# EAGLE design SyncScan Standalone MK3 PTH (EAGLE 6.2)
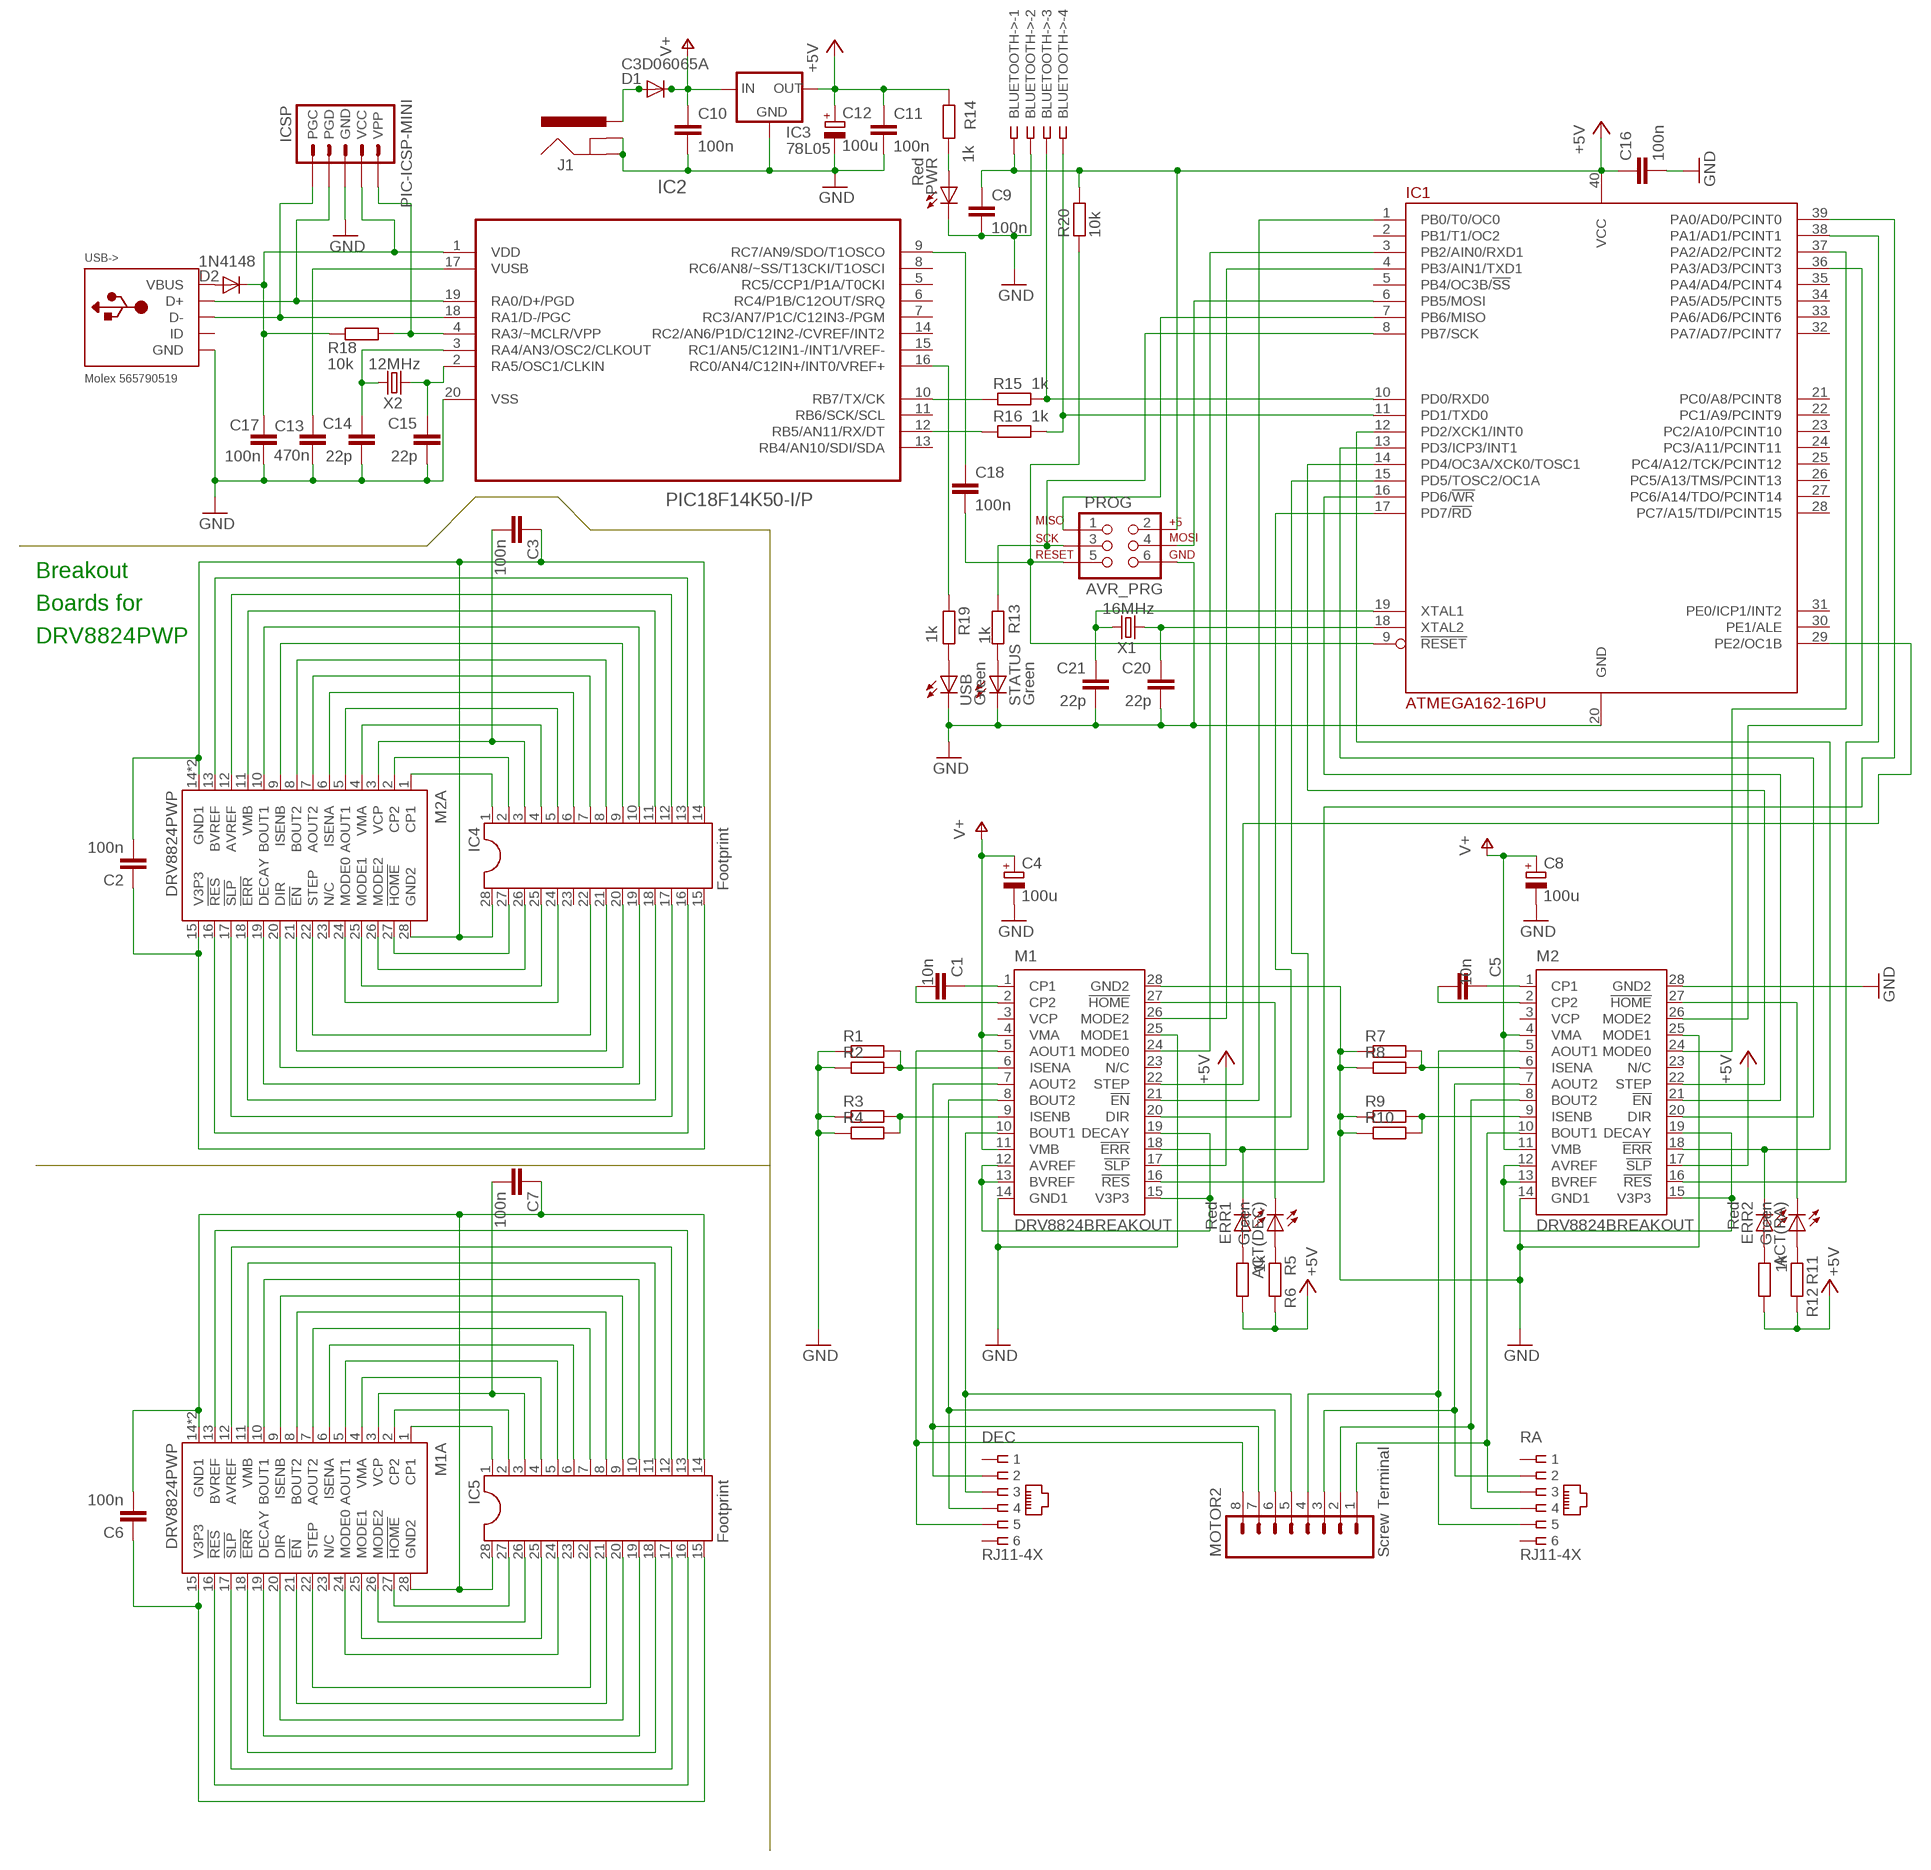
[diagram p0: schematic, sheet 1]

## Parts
ACT(DEC)  Green  LED3MM  [LED3MM]
ACT(RA)  Green  LED3MM  [LED3MM]
BLUETOOTH->  http://www.ebay.co.uk/itm/250991624201  SSW-104-02-S-S-RA  [SSW-104-02-S-S-RA]
C1  10n  C-EU025-024X044  [C025-024X044]
C2  100n  C-EUC0603K  [C0603K]
C3  100n  C-EUC0603K  [C0603K]
C4  100u  CPOL-EUE2.5-6  [E2,5-6]
C5  10n  C-EU025-024X044  [C025-024X044]
C6  100n  C-EUC0603K  [C0603K]
C7  100n  C-EUC0603K  [C0603K]
C8  100u  CPOL-EUE2.5-6  [E2,5-6]
C9  100n  C-EU025-024X044  [C025-024X044]
C10  100n  C-EU025-024X044  [C025-024X044]
C11  100n  C-EU025-024X044  [C025-024X044]
C12  100u  CPOL-EUE2.5-6  [E2,5-6]
C13  470n  C-EU025-024X044  [C025-024X044]
C14  22p  C-EU025-024X044  [C025-024X044]
C15  22p  C-EU025-024X044  [C025-024X044]
C16  100n  C-EU025-024X044  [C025-024X044]
C17  100n  C-EU025-024X044  [C025-024X044]
C18  100n  C-EU025-024X044  [C025-024X044]
C20  22p  C-EU025-024X044  [C025-024X044]
C21  22p  C-EU025-024X044  [C025-024X044]
D1  C3D06065A  BYW80  [TO220ACS]
D2  1N4148  DIODE1N4148  [DIODE-1N4148]
DEC  RJ11-4X  [RJ11-NO_SHIELD]
ERR1  Red  LED3MM  [LED3MM]
ERR2  Red  LED3MM  [LED3MM]
IC1  ATMEGA162-16PU  [DIL40]
IC2  PIC18F14K50-I/P  [DIL20]
IC3  78L05  V_REG_78XXTO-92  [TO-92]
IC4  Footprint  DIL28  [DIL28-6]
IC5  Footprint  DIL28  [DIL28-6]
ICSP  PIC-ICSP-MINI  [PIC-ICSP-MINI]
J1  POWER_JACKPTH  [POWER_JACK_PTH]
M1  DRV8824BREAKOUT  [DIL28-6]
M1A  DRV8824PWP  [HTSSOP28PWP]
M2  DRV8824BREAKOUT  [DIL28-6]
M2A  DRV8824PWP  [HTSSOP28PWP]
MOTOR2  Screw Terminal  M083.5MM-8  [SCREWTERMINAL-3.5MM-8]
PROG  AVR_PRG  AVR_SPI_PRG_6PTH  [2X3]
PWR  Red  LED3MM  [LED3MM]
R1  1.5R  R-EU_0309/12  [0309/12]
R2  1.5R  R-EU_0309/12  [0309/12]
R3  1.5R  R-EU_0309/12  [0309/12]
R4  1.5R  R-EU_0309/12  [0309/12]
R5  1k  R-EU_0204/7  [0204/7]
R6  1k  R-EU_0204/7  [0204/7]
R7  1.5R  R-EU_0309/12  [0309/12]
R8  1.5R  R-EU_0309/12  [0309/12]
R9  1.5R  R-EU_0309/12  [0309/12]
R10  1.5R  R-EU_0309/12  [0309/12]
R11  1k  R-EU_0204/7  [0204/7]
R12  1k  R-EU_0204/7  [0204/7]
R13  1k  R-EU_0204/7  [0204/7]
R14  1k  R-EU_0204/7  [0204/7]
R15  1k  R-EU_0204/7  [0204/7]
R16  1k  R-EU_0204/7  [0204/7]
R18  10k  R-EU_0204/7  [0204/7]
R19  1k  R-EU_0204/7  [0204/7]
R20  10k  R-EU_0204/7  [0204/7]
RA  RJ11-4X  [RJ11-NO_SHIELD]
STATUS  Green  LED3MM  [LED3MM]
USB  Green  LED3MM  [LED3MM]
USB->  Molex 565790519  USBMOLEX  [USB-MINIB-THM-MOLEX]
X1  16MHz  CRYSTALHC49US  [HC49US]
X2  12MHz  CRYSTALHC49US  [HC49US]

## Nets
3.3V-1: M1.12(AVREF) M1.13(BVREF) M1.15(V3P3) M1.19(DECAY)
3.3V-2: M2.12(AVREF) M2.13(BVREF) M2.15(V3P3) M2.19(DECAY)
!EN: IC4.21 M2A.21(!EN)
!EN1: IC5.21 M1A.21(!EN)
!EN-1: IC1.1(PB0/T0/OC0) M1.21(!EN)
!EN-2: IC1.16(PD6/!WR) M2.21(!EN)
!ERR: IC4.18 M2A.18(!ERR)
!ERR1: IC5.18 M1A.18(!ERR)
!ERR-1: ERR1.K(C) IC1.15(PD5/TOSC2/OC1A) M1.18(!ERR)
!ERR-2: ERR2.K(C) IC1.12(PD2/XCK1/INT0) M2.18(!ERR)
!HOME: IC4.27 M2A.27(!HOME)
!HOME1: IC5.27 M1A.27(!HOME)
!HOME-1: ACT(DEC).K(C) M1.27(!HOME)
!HOME-2: ACT(RA).K(C) M2.27(!HOME)
!RES: IC4.16 M2A.16(!RES)
!RES1: IC5.16 M1A.16(!RES)
!RST-1: IC1.39(PA0/AD0/PCINT0) M1.16(!RES)
!RST-2: IC1.38(PA1/AD1/PCINT1) M2.16(!RES)
!SLP: IC4.17 M2A.17(!SLP)
!SLP1: IC5.17 M1A.17(!SLP)
+5V: BLUETOOTH->.1 C9.1 C11.1 C12.+ C16.1 IC1.40(VCC) IC3.1(OUT) M1.17(!SLP) M2.17(!SLP) PROG.2 R5.2 R6.2 R11.2 R12.2 R14.1 R20.2
A1-1: DEC.5 M1.5(AOUT1) MOTOR2.8
A1-2: M2.5(AOUT1) MOTOR2.4 RA.5
A2-1: DEC.2 M1.7(AOUT2) MOTOR2.7
A2-2: M2.7(AOUT2) MOTOR2.3 RA.2
AOUT1: IC4.5 M2A.5(AOUT1)
AOUT2: IC4.7 M2A.7(AOUT2)
AOUT3: IC5.5 M1A.5(AOUT1)
AOUT4: IC5.7 M1A.7(AOUT2)
AVREF: IC4.12 M2A.12(AVREF)
AVREF1: IC5.12 M1A.12(AVREF)
AVROSC1: C21.1 IC1.19(XTAL1) X1.2
AVROSC2: C20.1 IC1.18(XTAL2) X1.1
B1-1: DEC.3 M1.10(BOUT1) MOTOR2.5
B1-2: M2.10(BOUT1) MOTOR2.1 RA.3
B2-1: DEC.4 M1.8(BOUT2) MOTOR2.6
B2-2: M2.8(BOUT2) MOTOR2.2 RA.4
BOUT1: IC4.10 M2A.10(BOUT1)
BOUT2: IC4.8 M2A.8(BOUT2)
BOUT3: IC5.8 M1A.8(BOUT2)
BOUT4: IC5.10 M1A.10(BOUT1)
BVREF: IC4.13 M2A.13(BVREF)
BVREF1: IC5.13 M1A.13(BVREF)
CP1: IC4.1 M2A.1(CP1)
CP1-1: C1.1 M1.1(CP1)
CP1-2: C5.1 M2.1(CP1)
CP2: IC4.2 M2A.2(CP2)
CP2-1: C1.2 M1.2(CP2)
CP2-2: C5.2 M2.2(CP2)
CP3: IC5.1 M1A.1(CP1)
CP4: IC5.2 M1A.2(CP2)
D+: IC2.19(RA0/D+/PGD) ICSP.4(PGD) USB->.D+
D-: IC2.18(RA1/D-/PGC) ICSP.5(PGC) USB->.D-
DECAY: IC4.19 M2A.19(DECAY)
DECAY1: IC5.19 M1A.19(DECAY)
DIR: IC4.20 M2A.20(DIR)
DIR1: IC5.20 M1A.20(DIR)
DIR-1: IC1.17(PD7/!RD) M1.20(DIR)
DIR-2: IC1.13(PD3/ICP3/INT1) M2.20(DIR)
GND: BLUETOOTH->.2 C4.- C8.- C9.2 C10.2 C11.2 C12.- C13.1 C14.2 C15.2 C16.2 C17.2 C20.2 C21.2 IC1.20(GND) IC2.20(VSS) IC3.2(GND) ICSP.3(GND) J1.GND J1.GNDBREAK M1.14(GND1) M1.25(MODE1) M1.28(GND2) M2.14(GND1) M2.25(MODE1) M2.28(GND2) PROG.6 PWR.K(C) R1.1 R2.1 R3.1 R4.1 R7.1 R8.1 R9.1 R10.1 STATUS.K(C) USB->.GND USB.K(C)
GND1: C6.2 C7.1 IC5.14 IC5.28 M1A.14(GND1) M1A.28(GND2) M1A.EXP(GND1)
GND2: C2.2 C3.1 IC4.14 IC4.28 M2A.14(GND1) M2A.28(GND2) M2A.EXP(GND1)
ISENA: IC4.6 M2A.6(ISENA)
ISENA1: IC5.6 M1A.6(ISENA)
ISENA-1: M1.6(ISENA) R1.2 R2.2
ISENA-2: M2.6(ISENA) R7.2 R8.2
ISENB: IC4.9 M2A.9(ISENB)
ISENB1: IC5.9 M1A.9(ISENB)
ISENB-1: M1.9(ISENB) R3.2 R4.2
ISENB-2: M2.9(ISENB) R9.2 R10.2
LED1: ERR1.A R6.1
LED2: ACT(DEC).A R5.1
LED3: ERR2.A R12.1
LED4: ACT(RA).A R11.1
M0-1: IC1.3(PB2/AIN0/RXD1) M1.24(MODE0)
M0-2: IC1.37(PA2/AD2/PCINT2) M2.24(MODE0)
M2-1: IC1.4(PB3/AIN1/TXD1) M1.26(MODE2)
M2-2: IC1.36(PA3/AD3/PCINT3) M2.26(MODE2)
MCLR: IC2.4(RA3/~MCLR/VPP) ICSP.1(VPP) R18.1
MISO: IC1.7(PB6/MISO) PROG.1
MODE0: IC4.24 M2A.24(MODE0)
MODE1: IC4.25 M2A.25(MODE1)
MODE2: IC4.26 M2A.26(MODE2)
MODE3: IC5.24 M1A.24(MODE0)
MODE4: IC5.25 M1A.25(MODE1)
MODE5: IC5.26 M1A.26(MODE2)
MOSI: IC1.6(PB5/MOSI) PROG.4
N$1: C18.1 IC2.9(RC7/AN9/SDO/T1OSCO)
PWRLED: PWR.A R14.2
RESET: C18.2 IC1.9(!RESET) PROG.5 R20.1
RX(BTH): BLUETOOTH->.4 IC1.11(PD1/TXD0) R16.1
RX(USB): IC2.12(RB5/AN11/RX/DT) R16.2
SCLK: IC1.8(PB7/SCK) PROG.3 R13.1
STATLED: R13.2 STATUS.A
STEP: IC4.22 M2A.22(STEP)
STEP1: IC5.22 M1A.22(STEP)
STEP-1: IC1.29(PE2/OC1B) M1.22(STEP)
STEP-2: IC1.14(PD4/OC3A/XCK0/TOSC1) M2.22(STEP)
TX(BTH): BLUETOOTH->.3 IC1.10(PD0/RXD0) R15.1
TX(USB): IC2.10(RB7/TX/CK) R15.2
USBLED: R19.1 USB.A
USBOSC1: C15.1 IC2.2(RA5/OSC1/CLKIN) X2.1
USBOSC2: C14.1 IC2.3(RA4/AN3/OSC2/CLKOUT) X2.2
USBSTAT: IC2.16(RC0/AN4/C12IN+/INT0/VREF+) R19.2
V3P1: C6.1 IC5.15 M1A.15(V3P3)
V3P3: C2.1 IC4.15 M2A.15(V3P3)
V+: C4.+ C8.+ C10.1 D1.C IC3.3(IN) M1.4(VMA) M1.11(VMB) M2.4(VMA) M2.11(VMB)
VBUS: D2.A USB->.VBUS
VCP: C3.2 IC4.3 M2A.3(VCP)
VCP1: C7.2 IC5.3 M1A.3(VCP)
VIN: D1.A J1.PWR
VMA: IC4.4 M2A.4(VMA)
VMA1: IC5.4 M1A.4(VMA)
VMB: IC4.11 M2A.11(VMB)
VMB1: IC5.11 M1A.11(VMB)
VPIC: C17.1 D2.C IC2.1(VDD) ICSP.2(VCC) R18.2
VUSB: C13.2 IC2.17(VUSB)
Unconnected: DEC.1 DEC.6 IC1.2(PB1/T1/OC2) IC1.5(PB4/OC3B/!SS) IC1.21(PC0/A8/PCINT8) IC1.22(PC1/A9/PCINT9) IC1.23(PC2/A10/PCINT10) IC1.24(PC3/A11/PCINT11) IC1.25(PC4/A12/TCK/PCINT12) IC1.26(PC5/A13/TMS/PCINT13) IC1.27(PC6/A14/TDO/PCINT14) IC1.28(PC7/A15/TDI/PCINT15) IC1.30(PE1/ALE) IC1.31(PE0/ICP1/INT2) IC1.32(PA7/AD7/PCINT7) IC1.33(PA6/AD6/PCINT6) IC1.34(PA5/AD5/PCINT5) IC1.35(PA4/AD4/PCINT4) IC2.5(RC5/CCP1/P1A/T0CKI) IC2.6(RC4/P1B/C12OUT/SRQ) IC2.7(RC3/AN7/P1C/C12IN3-/PGM) IC2.8(RC6/AN8/~SS/T13CKI/T1OSCI) IC2.11(RB6/SCK/SCL) IC2.13(RB4/AN10/SDI/SDA) IC2.14(RC2/AN6/P1D/C12IN2-/CVREF/INT2) IC2.15(RC1/AN5/C12IN1-/INT1/VREF-) IC4.23 IC5.23 M1.3(VCP) M1.23(N/C) M1A.23(N/C) M2.3(VCP) M2.23(N/C) M2A.23(N/C) RA.1 RA.6 USB->.ID

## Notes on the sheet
- Breakout
- Boards for
- DRV8824PWP

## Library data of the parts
ACT(DEC) ACT(RA) STATUS USB = led:LED: LED; MF: KINGBRIGHT; MPN: L-424GDT; OC_FARNELL: 1142496
BLUETOOTH-> = con-samtec:SSW-104-02-S-S: THROUGH-HOLE .025" SQ POST SOCKET Source: Samtec SSW.pdf; OC_FARNELL: unknown; OC_NEWARK: 11P9385
C1 C5 = resistor:C-EU: CAPACITOR, European symbol; MF: AVX; MPN: SR151C103KAR; OC_FARNELL: 1100380
C2 C3 C6 C7 = resistor:C-EU: CAPACITOR, European symbol; MF: KEMET; MPN: C0603C104K4RACTU; OC_FARNELL: 1414610
C4 C8 C12 = resistor:CPOL-EU: POLARIZED CAPACITOR, European symbol; MF: MULTICOMP; MPN: MCGPR25V107M6.3X11; OC_FARNELL: 9451188
C9-C11 C16-C18 = resistor:C-EU: CAPACITOR, European symbol; MF: AVX; MPN: SR205C104KAR; OC_FARNELL: 1100367
C13 = rcl:C-EU: CAPACITOR, European symbol; MF: KEMET; MPN: C320C474M5U5TA; OC_FARNELL: 1457660
C14 C15 C20 C21 = rcl:C-EU: CAPACITOR, European symbol; MF: AVX; MPN: SR151A220JAR; OC_FARNELL: 1100369
D1 = diode:BYW80: DIODE; MF: CREE; MPN: C3D06065A; OC_FARNELL: 1864928
D2 = SparkFun:DIODE: Diode; MF: MULTICOMP; MPN: 1N4148.; OC_FARNELL: 9565124
DEC RA = con-tycoelectronics:RJ11: CORCOM Modular RJ Jacks No Shield Source: www.tycoelectronics.com .. ENG_DS_1654001_1099_RJ_L_0507.pdf; MF: MH CONNECTORS; MPN: MHRJJ64NFRA; OC_FARNELL: 3938347; OC_NEWARK: 19R7022
ERR1 ERR2 PWR = led:LED: LED; MF: KINGBRIGHT; MPN: L-424HDT; OC_FARNELL: 1142499
IC1 = atmel:ATMEGA162: 8-bit RISC MICROCONTROLLER 16K Bytes internal flash program memory 1K Bytes internal SRAM Upto 64K Bytes optional external memory space 512 Bytes EEPROM Two 8-bit timers Two 16-bit timers Dual programmable serial USARTs Master/Slave serial SPI interface Source: ATMEGA162_DIP40.lbr; MF: ATMEL; MPN: ATMEGA162-16PU; OC_FARNELL: 9171169
IC2 = microchip:PIC18F14K50-I/P: USB Flash Microcontrollers; MF: MICROCHIP; MPN: PIC18F14K50-I/P; OC_FARNELL: 1648501; OC_NEWARK: 77M3103; PACKAGE: DIP-20; SUPPLIER: Microchip
IC3 = SparkFun:V_REG_78XX: Voltage Regulator Standard 7805 5V regulator. IGO (Input Ground Output). Spark Fun Electronics SKU : COM-00107; MF: FAIRCHILD SEMICONDUCTOR; MPN: LM78L05ACZX; OC_FARNELL: 1467367
IC4 IC5 = ic-package:DIL28: Dual In Line; MF: MULTICOMP; MPN: MC34735; OC_FARNELL: 1593421
ICSP = SparkFun:PIC-ICSP-MINI: PIC-ICSP-Mini Miniature 5-pin connection for temporary programming of PICs. Use this device in your design to save space. Program the PIC with this adapter Spark Fun Electronics SKU : BOB-00194; OC_FARNELL: unknown
J1 = SparkFun:POWER_JACK: Power Jack This is the standard 5.5mm barrel jack for power. The PTH is the most common, proven, reliable, footprint. All others are experimental. The Slot footprint only works if the mill layer is transmitted to the PCB fab house so be warned. Spark Fun Electronics SKU : PRT-00119. Mating wall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; MF: MULTICOMP; MPN: MJ-179PH; OC_FARNELL: 1737246
M1 M2 = texas:DRV8824; MF: MULTICOMP; MPN: MC-2227-28-06-F1; OC_FARNELL: 1182591
M1A M2A = texas:DRV8824; MF: TEXAS INSTRUMENTS; MPN: DRV8824PWP; OC_FARNELL: 1815786
MOTOR2 = SparkFun:M08: Header 8 Standard 8-pin 0.1" header. Use with straight break away headers (SKU : PRT-00116), right angle break away headers (PRT-00553), swiss pins (PRT-00743), machine pins (PRT-00117), and female headers (PRT-00115).; MF: LUMBERG; MPN: KRMC 08; OC_FARNELL: 1217307
PROG = SparkFun:AVR_SPI_PRG_6: AVR ISP 6 Pin This is the reduced ISP connector for AVR programming. Common on Arduino. This footprint will take up less PCB space and can be used with a 10-pin to 6-pin adapter such as SKU: BOB-08508; MF: TE CONNECTIVITY / AMP; MPN: 826632-3; OC_FARNELL: 3418492
R1-R4 R7-R10 = resistor:R-EU_: RESISTOR, European symbol; MF: WELWYN; MPN: MFP1-1R5 JI; OC_FARNELL: 1565361
R5 R6 R11 R12 = resistor:R-EU_: RESISTOR, European symbol; MF: MULTICOMP; MPN: MF12 1K; OC_FARNELL: 9342400
R13 R14 R19 = rcl:R-EU_: RESISTOR, European symbol; MF: MULTICOMP; MPN: MF12 1K; OC_FARNELL: 9342400
R15 R16 = SmartPrj:R-EU_: RESISTOR, European symbol; MF: MULTICOMP; MPN: MF12 1K; OC_FARNELL: 9342400
R18 R20 = rcl:R-EU_: RESISTOR, European symbol; MF: MULTICOMP; MPN: MF12 10K; OC_FARNELL: 9342419
USB-> = adafruit:USB: USB Connectors USBMINIB - Surface Mount Female Mini-B USB Connector 4UConnector: 06564 By microbuilder.eu Thru-hole RA Female Mini-B USB Connector 4UConnector: 18732 By ladyada.net; MF: MOLEX; MPN: 565790519; OC_FARNELL: 1125347
X1 = SparkFun:CRYSTAL: Crystals; MF: TXC; MPN: 9B-16.000MEEJ-B; OC_FARNELL: 1842217
X2 = SparkFun:CRYSTAL: Crystals; MF: TXC; MPN: 9B-12.000MAAJ-B; OC_FARNELL: 1842203

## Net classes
1 power: width 0.61 mm, drill 0.711 mm, clearance 0.203 mm
2 gnd: width 0.305 mm, drill 0.711 mm, clearance 0.203 mm
3 usbvcc: width 0.508 mm, drill 0.711 mm, clearance 0.203 mm

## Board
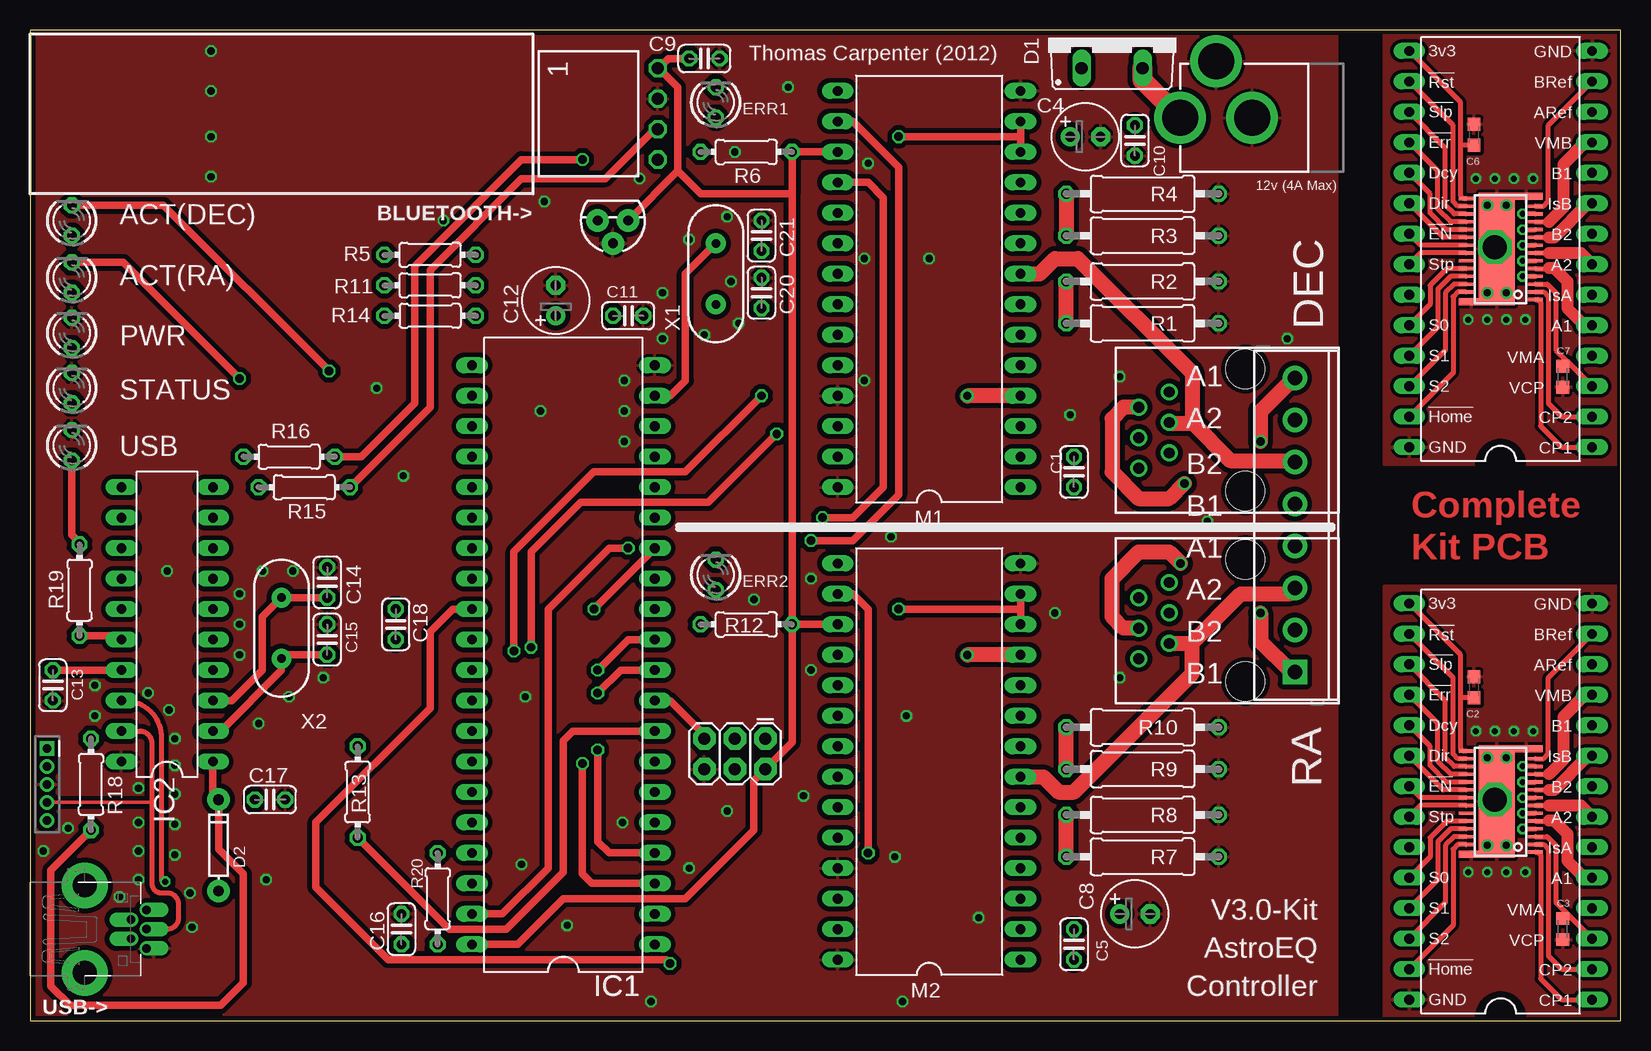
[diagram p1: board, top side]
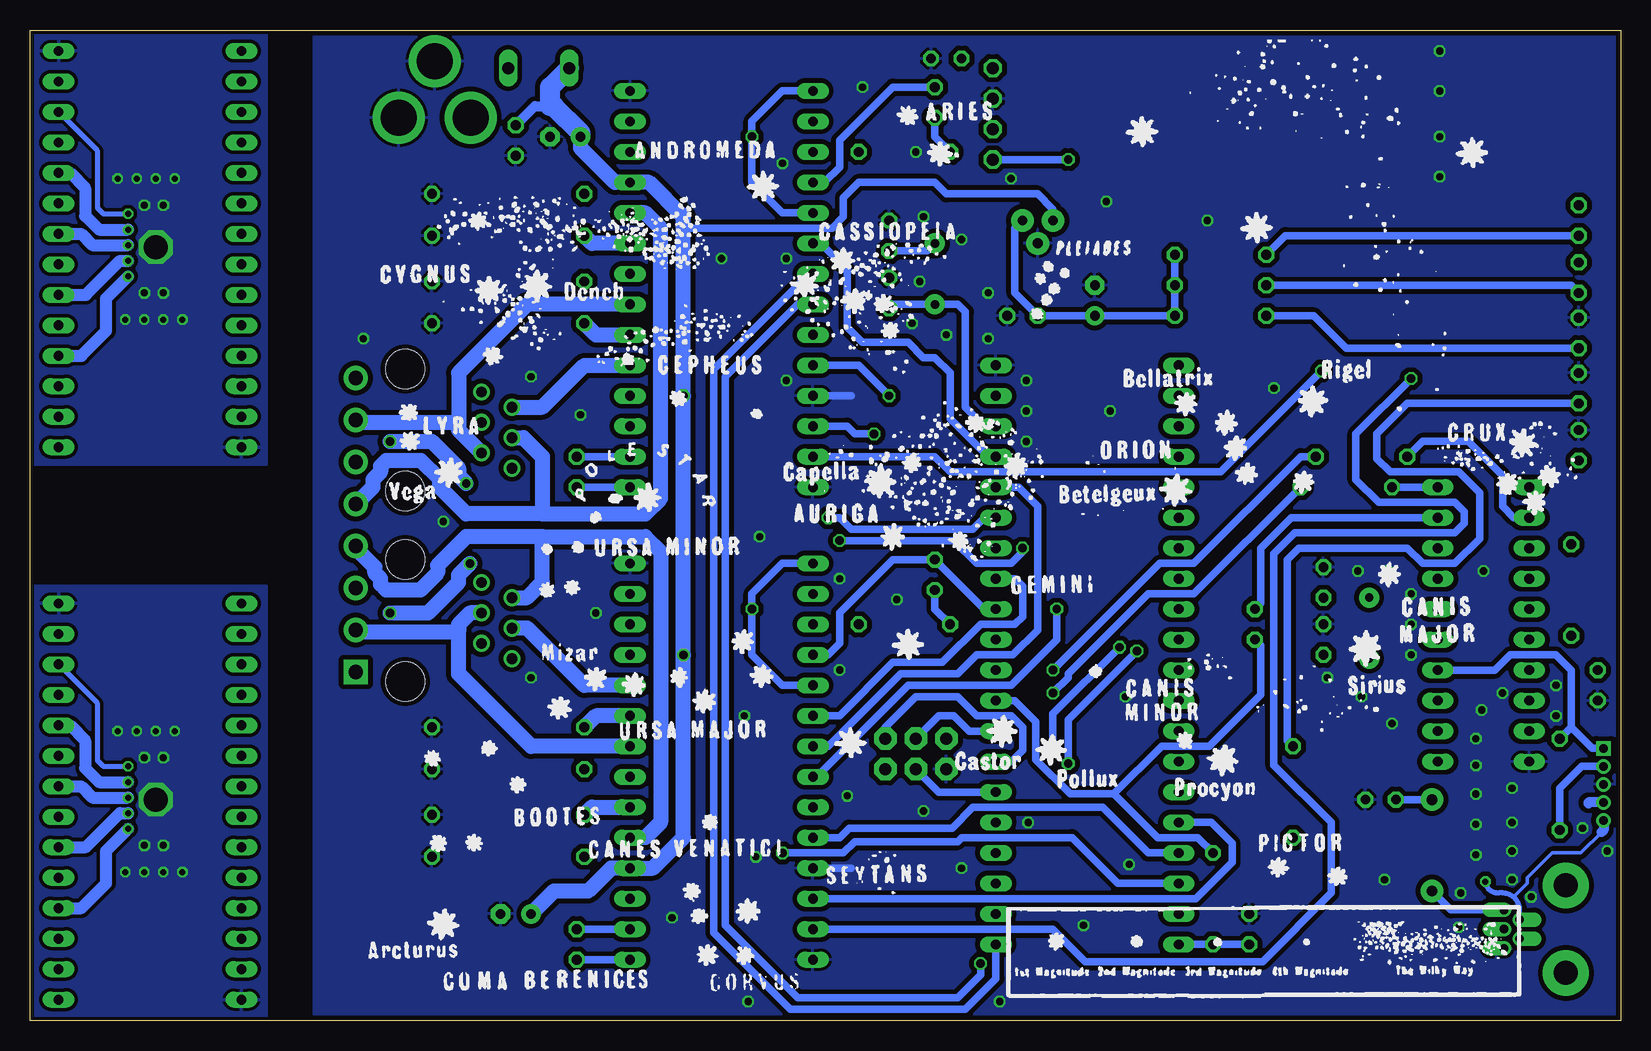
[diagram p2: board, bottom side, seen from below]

Size 132.56 x 82.55 mm. Coordinates in mm from the lower left corner, seen from the top.
Outline: 0,82.55 0,0 132.56,0 132.56,82.55 0,82.55
Copper layers (1*16): Top 0.035mm / dielectric 1.5mm / Bottom 0.035mm
Design rules: minimum track width 0.2mm, minimum drill 0.49mm, track to track 0.2mm, track to pad 0.2mm, pad to pad 0.2mm, via to via 0.2mm, smd to smd 0mil, copper to edge 10mil, drill to drill 0.2mm, minimum pad ring 10mil, minimum via ring 7mil, stop-mask expansion 0.125mm, vias tented up to drill 0mil, thermal gap 10mil
tRestrict: area 120.9,0.3 to 124.2,2; area 120.9,46.4 to 124.2,48

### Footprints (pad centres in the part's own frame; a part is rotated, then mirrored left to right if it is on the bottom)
LED3MM = drill 0.813 octagon: A -1.27,0; K 1.27,0
SSW-104-02-S-S-RA = drill 1 pad 1.5 octagon: 1 -3.81,1.524; 2 -1.27,1.524; 3 1.27,1.524; 4 3.81,1.524
C025-024X044 = drill 0.813 octagon: 1 -1.27,0; 2 1.27,0
C0603K = smd 1.05 x 1.08: 1 -0.875,0; 2 0.875,0
E2,5-6 = drill 0.813 pad 1.6: + -1.27,0 | drill 0.813 pad 1.6 octagon: - 1.27,0
TO220ACS = drill 1.016 long: A 2.54,-2.54; C -2.54,-2.54
DIODE-1N4148 = drill 0.9 pad 1.88: A -3.81,0; C 3.81,0
RJ11-NO_SHIELD = drill 0.9 pad 1.4: 1 -3.175,8.89; 2 -1.905,6.35; 3 -0.635,8.89; 4 0.635,6.35; 5 1.905,8.89; 6 3.175,6.35 | hole 3.251: -5.08,0; 5.08,0
DIL40 = drill 0.813 long: 1 -24.13,-7.62; 2 -21.59,-7.62; 3 -19.05,-7.62; 4 -16.51,-7.62; 5 -13.97,-7.62; 6 -11.43,-7.62; 7 -8.89,-7.62; 8 -6.35,-7.62; 9 -3.81,-7.62; 10 -1.27,-7.62; 11 1.27,-7.62; 12 3.81,-7.62; 13 6.35,-7.62; 14 8.89,-7.62; 15 11.43,-7.62; 16 13.97,-7.62; 17 16.51,-7.62; 18 19.05,-7.62; 19 21.59,-7.62; 20 24.13,-7.62; 21 24.13,7.62; 22 21.59,7.62; 23 19.05,7.62; 24 16.51,7.62; 25 13.97,7.62; 26 11.43,7.62; 27 8.89,7.62; 28 6.35,7.62; 29 3.81,7.62; 30 1.27,7.62; 31 -1.27,7.62; 32 -3.81,7.62; 33 -6.35,7.62; 34 -8.89,7.62; 35 -11.43,7.62; 36 -13.97,7.62; 37 -16.51,7.62; 38 -19.05,7.62; 39 -21.59,7.62; 40 -24.13,7.62
DIL20 = drill 0.813 long: 1 -3.81,11.43; 2 -3.81,8.89; 3 -3.81,6.35; 4 -3.81,3.81; 5 -3.81,1.27; 6 -3.81,-1.27; 7 -3.81,-3.81; 8 -3.81,-6.35; 9 -3.81,-8.89; 10 -3.81,-11.43; 11 3.81,-11.43; 12 3.81,-8.89; 13 3.81,-6.35; 14 3.81,-3.81; 15 3.81,-1.27; 16 3.81,1.27; 17 3.81,3.81; 18 3.81,6.35; 19 3.81,8.89; 20 3.81,11.43
TO-92 = drill 0.813 pad 1.88: 1 -1.27,0; 2 0,1.905; 3 1.27,0
DIL28-6 = drill 0.813 long: 1 -16.51,-7.62; 2 -13.97,-7.62; 3 -11.43,-7.62; 4 -8.89,-7.62; 5 -6.35,-7.62; 6 -3.81,-7.62; 7 -1.27,-7.62; 8 1.27,-7.62; 9 3.81,-7.62; 10 6.35,-7.62; 11 8.89,-7.62; 12 11.43,-7.62; 13 13.97,-7.62; 14 16.51,-7.62; 15 16.51,7.62; 16 13.97,7.62; 17 11.43,7.62; 18 8.89,7.62; 19 6.35,7.62; 20 3.81,7.62; 21 1.27,7.62; 22 -1.27,7.62; 23 -3.81,7.62; 24 -6.35,7.62; 25 -8.89,7.62; 26 -11.43,7.62; 27 -13.97,7.62; 28 -16.51,7.62
PIC-ICSP-MINI = drill 0.7 square: 1 -3,0 | drill 0.7: 2 -1.5,0; 3 0,0; 4 1.5,0; 5 3,0
POWER_JACK_PTH = drill 2.997 pad 4.318: GND 0,7.7; GNDBREAK 4.7,10.7; PWR 0,13.7
DIL28-6' = drill 0.813 pad 1.2 long: 1 -16.51,-7.62; 2 -13.97,-7.62; 3 -11.43,-7.62; 4 -8.89,-7.62; 5 -6.35,-7.62; 6 -3.81,-7.62; 7 -1.27,-7.62; 8 1.27,-7.62; 9 3.81,-7.62; 10 6.35,-7.62; 11 8.89,-7.62; 12 11.43,-7.62; 13 13.97,-7.62; 14 16.51,-7.62; 15 16.51,7.62; 16 13.97,7.62; 17 11.43,7.62; 18 8.89,7.62; 19 6.35,7.62; 20 3.81,7.62; 21 1.27,7.62; 22 -1.27,7.62; 23 -3.81,7.62; 24 -6.35,7.62; 25 -8.89,7.62; 26 -11.43,7.62; 27 -13.97,7.62; 28 -16.51,7.62
HTSSOP28PWP = smd 0.27 x 1.2: 1 -4.21,-2.9; 2 -3.575,-2.9; 3 -2.925,-2.9; 4 -2.275,-2.9; 5 -1.625,-2.9; 6 -0.975,-2.9; 7 -0.325,-2.9; 8 0.325,-2.9; 9 0.975,-2.9; 10 1.625,-2.9; 11 2.275,-2.9; 12 2.925,-2.9; 13 3.575,-2.9; 15 4.21,2.9; 16 3.575,2.9; 17 2.925,2.9; 18 2.275,2.9; 19 1.625,2.9; 20 0.975,2.9; 21 0.325,2.9; 22 -0.325,2.9; 23 -0.975,2.9; 24 -1.625,2.9; 25 -2.275,2.9; 26 -2.925,2.9; 27 -3.575,2.9 | smd 0.61 x 2.735: 14 4.395,-2.132 | smd 0.61 x 2.1: 28 -4.395,2.45 | smd 9.4 x 3: EXP 0,0.318
SCREWTERMINAL-3.5MM-8 = drill 1.2 pad 2.032 square: 1 0,0 | drill 1.2 pad 2.032: 2 3.5,0; 3 7,0; 4 10.5,0; 5 14,0; 6 17.5,0; 7 21,0; 8 24.5,0
2X3 = drill 1.016 pad 1.88 octagon: 1 0,0; 2 0,2.54; 3 2.54,0; 4 2.54,2.54; 5 5.08,0; 6 5.08,2.54
0309/12 = drill 0.813 octagon: 1 -6.35,0; 2 6.35,0
0204/7 = drill 0.813 octagon: 1 -3.81,0; 2 3.81,0
USB-MINIB-THM-MOLEX = drill 0.7 offset: D+ 0,9.72; D- -0.8,8.42; GND 1.6,9.72; ID 0.8,8.42; VBUS -1.6,9.72 | drill 2 pad 3.81: GND1 -3.65,4.57; GND4 3.65,4.57
HC49US = drill 0.7 pad 1.651: 1 -2.54,0; 2 2.54,0

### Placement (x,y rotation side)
ACT(DEC)  3.49,66.67 90 top
ACT(RA)  3.49,61.91 90 top
BLUETOOTH->  50.8,75.56 270 top
C1  87,45.72 90 top
C2  120.33,27.78 90 top
C3  127.71,7.62 90 top
C4  87.95,73.66 0 top
C5  87,6.35 90 top
C6  120.33,73.82 90 top
C7  127.71,53.66 90 top
C8  92.08,8.89 0 top
C9  56.2,80.17 0 top
C10  92.08,73.34 270 top
C11  49.85,58.74 0 top
C12  43.81,60.01 90 top
C13  1.91,27.94 90 top
C14  24.77,36.51 90 top
C15  24.77,31.75 90 top
C16  30.96,7.62 90 top
C17  20,18.41 0 top
C18  30.48,33.02 270 top
C20  60.96,60.64 90 top
C21  60.96,65.41 90 top
D1  90.17,81.92 0 top
D2  15.72,14.61 90 top
DEC  101.28,49.21 90 top
ERR1  57.15,76.52 90 top
ERR2  57.15,37.15 90 top
IC1  44.45,30.48 90 top
IC2  11.43,33.02 180 top
IC3  48.58,66.67 180 top
IC4  122.56,18.26 90 top
IC5  122.56,64.29 90 top
ICSP  1.43,19.68 270 top
J1  109.54,75.25 90 top
M1  DRV8824BREAKOUT  [DIL28-6']  74.93,60.96 90 top
M1A  122.56,64.29 90 top
M2  DRV8824BREAKOUT  [DIL28-6']  74.93,21.59 90 top
M2A  122.56,18.26 90 top
MOTOR2  105.41,29.05 90 top
PROG  61.28,23.5 180 top
PWR  3.49,57.31 90 top
R1  92.71,58.1 180 top
R2  92.71,61.59 180 top
R3  92.71,65.41 180 top
R4  92.71,68.9 180 top
R5  33.34,63.82 0 top
R6  59.69,72.39 0 top
R7  92.71,13.65 180 top
R8  92.71,17.14 180 top
R9  92.71,20.95 180 top
R10  92.71,24.45 180 top
R11  33.34,61.28 0 top
R12  59.69,33.02 0 top
R13  27.3,19.05 90 top
R14  33.34,58.74 180 top
R15  22.86,44.45 180 top
R16  21.59,46.99 180 top
R18  5.08,19.68 270 top
R19  4.13,35.88 270 top
R20  33.97,10.16 270 top
RA  101.28,33.34 90 top
STATUS  3.49,52.7 90 top
USB  3.49,47.94 90 top
USB->  0,7.62 270 top
X1  57.15,62.23 90 top
X2  20.95,32.7 90 top

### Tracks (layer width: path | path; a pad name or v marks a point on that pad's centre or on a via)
3.3V-1  (via drill 0.7)
  Top 0.61: 82.55,73.66 M1.12 | M1.13 82.55,73.66 | 82.55,73.66 v72.39,73.66
  Bottom 0.61: M1.15 69.85,77.47 72.39,74.93 v72.39,73.66 72.39,69.85 69.85,67.31 M1.19
3.3V-2  (via drill 0.7)
  Top 0.61: M2.13 82.55,34.29 | 82.55,34.29 v72.39,34.29 | M2.12 82.55,34.29
  Bottom 0.61: M2.15 69.85,38.1 72.39,35.56 v72.39,34.29 72.39,30.48 69.85,27.94 M2.19
!EN
  Top 0.406: M2A.21 115.88,18.58 IC4.21
!EN1
  Top 0.406: M1A.21 115.88,64.62 IC5.21
!EN-1
  Bottom 0.61: M1.21 67.63,62.23 75.56,54.29 75.56,7.3 69.22,0.95 54.61,0.95 52.07,3.49 IC1.1
!EN-2
  Bottom 0.61: M2.21 66.04,22.86 60.01,28.89 55.24,28.89 53.66,30.48 50.64,30.48 48.58,32.54 48.58,42.86 50.16,44.45 IC1.16
!ERR
  Top 0.406: M2A.18 118.38,20.53 117.32,21.59 117.32,24.77 IC4.18
!ERR1
  Top 0.406: M1A.18 118.38,66.57 117.32,67.63 117.32,70.8 IC5.18
!ERR-1  (via drill 0.7)
  Top 0.61: M1.18 69.85,69.85 71.12,68.58 71.12,44.45 68.58,41.91 v66.04,41.91
  Bottom 0.61: M1.18 66.36,69.85 65.09,71.12 65.09,73.34 60.64,77.79 ERR1.K | v66.04,41.91 65.09,41.91 64.14,40.96 53.98,40.96 53.02,41.91 IC1.15
!ERR-2
  Bottom 0.61: M2.18 66.04,30.48 65.09,31.43 65.09,33.97 60.64,38.42 ERR2.K 53.02,34.29 IC1.12
!HOME
  Top 0.406: M2A.27 118.98,14.68 118.59,14.29 118.59,7.94 IC4.27
!HOME1
  Top 0.406: M1A.27 118.98,60.72 118.59,60.33 118.59,53.98 IC5.27
!HOME-1  (via drill 0.7)
  Top 0.61: ACT(DEC).K 11.11,67.94 v24.92,54.13
  Bottom 0.61: M1.27 57.15,46.99 55.88,45.72 33.34,45.72 v24.92,54.13
!HOME-2  (via drill 0.7)
  Top 0.61: ACT(RA).K 7.78,63.18 v17.46,53.5
  Bottom 0.61: M2.27 47.31,7.62 44.61,4.92 29.84,4.92 24.13,10.64 24.13,16.51 28.89,21.27 28.89,38.89 27.15,40.64 13.81,40.64 13.02,41.43 13.02,42.39 13.81,43.18 20.16,43.18 22.07,45.09 22.07,48.9 v17.46,53.5
!RES
  Top 0.406: M2A.16 118.98,21.83 118.59,22.23 118.59,28.57 IC4.16
!RES1
  Top 0.406: M1A.16 118.98,67.87 118.59,68.26 118.59,74.61 IC5.16
!RST-1  (via drill 0.7)
  Top 0.61: M1.16 68.58,74.93 72.39,71.12 72.39,43.81 68.58,40.01 v65.09,40.01 | IC1.39 39.37,8.89 43.18,12.7 43.18,34.29 48.26,39.37 v49.85,39.37
  Bottom 0.61: v65.09,40.01 55.56,40.01 53.66,38.1 50.8,38.1 49.85,39.05 v49.85,39.37
!RST-2  (via drill 0.7)
  Top 0.61: M2.16 68.58,35.56 69.85,34.29 v69.85,13.97
  Bottom 0.61: v69.85,13.97 64.77,13.97 63.82,14.92 55.24,14.92 54.93,15.24 45.72,15.24 41.91,11.43 IC1.38
!SLP
  Top 0.406: M2A.17 118.68,21.18 117.95,21.91 117.95,26.67 IC4.17
!SLP1
  Top 0.406: M1A.17 118.68,67.22 117.95,67.94 117.95,72.71 IC5.17
+5V
  Top 0.61: R12.2 63.5,68.9 | M1.17 R6.2 63.5,68.9 | M2.17 R12.2 | R12.2 63.5,23.18 PROG.2 60.33,20 60.33,15.88 54.61,10.16 44.45,10.16 40.64,6.35 IC1.40 | IC3.1 53.98,70.8 | 53.98,70.8 55.88,68.9 63.5,68.9 | 53.98,70.8 53.98,77.79 52.39,79.38 | C9.1 53.18,80.17 52.39,79.38 | 52.39,79.38 BLUETOOTH->.1
  Bottom 0.61: IC1.40 R20.2 C16.1 | IC3.1 50.48,66.04 50.48,60.64 C11.1 C12.+ R14.1 R11.2 R5.2
A1-1  (via drill 0.7)
  Top 1.27: MOTOR2.8 105.41,53.34 105.09,53.34 102.55,50.8 v102.55,48.26 | DEC.5 91.12,51.12 90.17,50.16 90.17,45.72 92.39,43.5 94.93,43.5 v96.2,44.77
  Bottom 1.27: M1.5 86.36,54.61 89.85,51.12 DEC.5 | v102.55,48.26 99.06,48.26 96.84,46.04 96.84,45.4 v96.2,44.77
A1-2
  Bottom 1.27: 89.85,40.32 89.85,36.51 91.12,35.24 RA.5 | 89.85,40.32 81.28,40.32 80.01,39.05 80.01,16.51 81.28,15.24 M2.5 | 89.85,40.32 96.2,40.32 98.58,37.94 98.58,37.33 100.03,35.88 102.87,35.88 103.35,36.35 103.35,36.83 103.82,37.31 103.82,37.78 105.41,39.37 MOTOR2.4
A2-1
  Bottom 1.27: M1.7 91.12,59.69 96.84,53.98 96.84,49.85 | 96.84,49.85 96.84,49.21 DEC.2 | 96.84,49.85 105.41,49.85 105.45,49.89 105.45,50.01 MOTOR2.7
A2-2
  Top 1.27: M2.7 84.45,20.32 85.72,19.05 87,19.05 96.84,28.89 96.84,31.43 | 96.84,31.43 96.84,31.5 100.9,35.56 104.92,35.56 MOTOR2.3 | RA.2 96.84,31.43
AOUT1
  Top 0.406: 129.54,11.91 IC4.5 | M2A.5 126.56,16.63 126.59,16.66
  Top 1.016: 129.54,11.91 128.11,13.34 128.11,15.56 127,16.67 126.99,16.66 126.59,16.66
AOUT2
  Top 0.406: M2A.7 126.58,17.93 126.59,17.94
  Top 1.016: 126.59,17.94 129.23,17.94 129.23,17.93 IC4.7
AOUT3
  Top 0.406: 129.54,57.94 IC5.5 | M1A.5 126.56,62.67 126.59,62.7
  Top 1.016: 129.54,57.94 128.11,59.37 128.11,61.59 127.01,62.7 126.59,62.7
AOUT4
  Top 0.406: M1A.7 126.58,63.97 126.59,63.98
  Top 1.016: 126.59,63.98 129.23,63.98 129.23,63.97 IC5.7
AVREF  (via drill 0.5)
  Top 0.406: M2A.12 124.39,21.18 v124.38,21.19
  Bottom 0.406: IC4.12 126.92,26.43 126.92,21.67 126.43,21.18 124.39,21.18 v124.38,21.19
AVREF1  (via drill 0.5)
  Top 0.406: M1A.12 124.39,67.22 v124.38,67.23
  Bottom 0.406: IC5.12 126.92,72.47 126.92,67.71 126.43,67.22 124.39,67.22 v124.38,67.23
AVROSC1
  Top 0.61: IC1.19 53.34,52.07 54.61,53.34 54.61,62.23 X1.2
  Bottom 0.61: C21.1 57.78,64.14 X1.2
AVROSC2
  Bottom 0.61: IC1.18 53.02,49.53 54.61,51.12 54.61,59.05 55.24,59.69 X1.1 60.64,59.69 C20.1
B1-1
  Bottom 1.27: 89.85,42.23 89.85,46.99 91.44,48.58 DEC.3 | 89.85,42.23 81.28,42.23 80.01,43.5 80.01,66.04 81.28,67.31 M1.10 | 89.85,42.23 96.2,42.23 98.42,44.45 98.42,45.12 99.98,46.67 102.87,46.67 103.35,46.2 103.35,45.72 103.98,45.09 103.98,44.45 105.38,43.05 MOTOR2.5
B1-2  (via drill 0.7)
  Top 1.27: v95.89,38.1 94.93,39.05 92.39,39.05 90.17,36.83 90.17,33.66 91.12,32.7 RA.3 | v102.55,33.97 102.55,31.59 105.09,29.05 MOTOR2.1
  Bottom 1.27: M2.10 86.36,27.94 91.12,32.7 RA.3 | v102.55,33.97 99.38,33.97 96.84,36.51 96.84,37.15 v95.89,38.1
B2-1
  Top 1.27: M1.8 84.14,62.23 85.41,63.5 87.31,63.5 96.84,53.98 96.84,49.85 | 96.84,49.85 96.84,49.78 95,49.78 DEC.4 | 96.84,49.85 100.01,46.67 105.41,46.67 MOTOR2.6
B2-2
  Bottom 1.27: M2.8 90.81,22.86 96.84,28.89 96.84,32.38 | 96.84,32.38 105.24,32.38 MOTOR2.2 | RA.4 95.89,33.97 96.84,33.02 96.84,32.38
BOUT1  (via drill 0.5)
  Top 0.406: v124.38,19.88 M2A.10
  Bottom 1.016: IC4.10 129.22,24.61 127.95,23.34 127.95,21.03 126.8,19.88 v124.39,19.88 v124.38,19.88
BOUT2  (via drill 0.5)
  Top 0.406: v124.38,18.58 M2A.8
  Bottom 1.016: IC4.8 128.31,19.53 127.36,18.58 v124.38,18.58
BOUT3  (via drill 0.5)
  Top 0.406: v124.38,64.62 M1A.8
  Bottom 1.016: IC5.8 128.31,65.56 127.36,64.62 v124.38,64.62
BOUT4  (via drill 0.5)
  Top 0.406: v124.38,65.91 v124.38,65.92 M1A.10
  Bottom 1.016: IC5.10 129.22,70.64 127.95,69.37 127.95,67.07 126.8,65.92 v124.39,65.92 v124.38,65.91
BVREF
  Top 0.406: M2A.13 126.13,21.83 126.52,22.23 126.52,28.57 IC4.13
BVREF1
  Top 0.406: M1A.13 126.13,67.87 126.52,68.26 126.52,74.61 IC5.13
CP1
  Top 0.406: M2A.1 125.65,14.05 125.89,13.81 125.89,3.49 127.64,1.75 IC4.1
CP1-1
  Bottom 0.61: C1.1 M1.1
CP1-2
  Bottom 0.61: C5.1 M2.1
CP2
  Top 0.406: M2A.2 126.13,14.68 126.52,14.29 126.52,5.4 127.64,4.29 IC4.2
CP2-1
  Bottom 0.61: C1.2 M1.2
CP2-2
  Bottom 0.61: C5.2 M2.2
CP3
  Top 0.406: M1A.1 125.65,60.08 125.89,59.85 125.89,49.53 127.64,47.78 IC5.1
CP4
  Top 0.406: M1A.2 126.13,60.72 126.52,60.33 126.52,51.44 127.64,50.32 IC5.2
D+
  Top 0.279: ICSP.4 10.16,18.18 10.16,18.26
  Top 0.406: USB->.D+ 11.43,7.62 arc90 12.38,8.57 12.38,9.68 arc90 11.43,10.64 10.95,10.64 arc-90 10.16,11.43 10.16,18.26 10.16,23.02 arc90 9.21,24.13 IC2.19
  Bottom 0.813: ICSP.4 2.7,18.18 2.7,18.1
D-  (via drill 0.5)
  Top 0.406: IC2.18 7.94,26.67 arc-90 10.95,23.5 10.95,11.75 arc90 11.11,11.59 v11.27,11.59
  Bottom 0.279: 1.59,15.72 3.33,13.97 5.71,13.97 7.78,11.91 7.78,11.43 8.89,10.32 arc90 9.05,10.32 arc-46 9.84,10.64
  Bottom 0.406: USB->.D- 8.42,9.21 arc-90 9.84,10.64 10.16,10.64 arc90 v11.27,11.59
  Bottom 0.813: ICSP.5 1.43,15.88 1.59,15.72
DECAY
  Top 0.406: M2A.19 118.07,19.88 116.68,21.27 116.68,22.86 IC4.19
DECAY1
  Top 0.406: M1A.19 118.07,65.92 116.68,67.31 116.68,68.9 IC5.19
DIR
  Top 0.406: M2A.20 117.77,19.23 IC4.20
DIR1
  Top 0.406: M1A.20 117.77,65.27 IC5.20
DIR-1
  Bottom 0.61: IC1.17 52.7,46.99 55.88,50.16 55.88,53.98 57.15,55.24 58.1,55.24 59.37,56.52 63.18,56.52 64.45,57.78 64.45,62.55 66.67,64.77 M1.20
DIR-2
  Bottom 0.61: M2.20 65.09,25.4 60.64,29.84 56.52,29.84 53.34,33.02 50.48,33.02 49.85,33.66 49.85,36.2 50.48,36.83 IC1.13
GND  (via drill 0.6)
  Bottom 0.61: M1.25 64.14,52.07 | M2.25 64.14,12.7
  other vias: 58.1,17.46 41.27,26.99 42.55,50.8 21.59,26.99 19.37,37.47 90.81,53.66 17.46,35.56 49.53,50.8 49.53,48.26 49.53,53.34 34.45,66.67 15.08,70.33 15.08,80.8 15.08,77.47 65.09,36.83 63.18,77.79 52.7,56.83 58.1,66.99 72.07,13.65 24.45,28.57 21.91,37.47 56.2,57.15 17.46,30.48 17.46,33.02 31.11,45.4 19.68,11.75 19.05,24.77 60.33,35.08 40.96,13.02 11.43,37.47 73.03,25.4 51.75,1.59 58.74,72.39 5.4,27.94 50.8,70.17 15.08,73.66 72.71,1.59 28.89,52.7 42.86,68.26 12.06,18.89 9.05,14.13 12.06,13.81 12.06,23.5 9.05,11.75 13.49,7.78 7.46,10.32 12.06,21.27 13.34,10.64 11.59,25.88 52.7,60.64 58.42,61.59 79.06,8.57 5.4,25.4 54.93,65.09 12.06,16.35 9.05,16.51 86.68,50.48 85.41,33.97 9.84,27.3 49.37,16.51 44.77,7.94 98.11,41.59 64.45,18.73 104.78,56.83 90.81,28.57 71.75,40.32 69.53,53.34 65.09,29.21 59.05,58.1 69.85,71.44 69.53,63.5 74.93,63.5 1.11,14.13 9.05,19.37 3.17,16.03 54.93,12.7
  pour Bottom (isolate 0.406): 0,82.55 108.9,82.55 108.9,0 0,0
  pour Top (isolate 0.406, rank 2): 0,82.55 108.9,82.55 108.9,0 0,0
GND1  (via drill 0.5, 0.6, 2)
  other vias: 119.86,58.42 121.44,58.42 123.03,58.42 124.62,58.42 121.44,60.64 123.03,60.64 122.08,64.45 121.44,67.94 123.03,67.94 125.25,70.17 123.67,70.17 122.08,70.17 120.49,70.17
  pour Bottom (isolate 0.305): 112.87,46.35 132.56,46.35 132.56,82.55 112.87,82.55
  pour Top (isolate 0.305, rank 2): 112.87,46.35 132.56,46.35 132.56,82.55 112.87,82.55
GND2  (via drill 0.5, 0.6, 2)
  other vias: 122.08,18.41 121.44,14.61 123.03,14.61 119.86,12.38 121.44,12.38 123.03,12.38 124.62,12.38 120.49,24.13 122.08,24.13 123.67,24.13 125.25,24.13 121.44,21.91 123.03,21.91
  pour Top (isolate 0.305, rank 2): 112.87,0 132.56,0 132.56,36.2 112.87,36.2
  pour Bottom (isolate 0.305): 112.87,0 132.56,0 132.56,36.2 112.87,36.2
ISENA  (via drill 0.5)
  Top 0.406: v124.38,17.27 v124.38,17.28 M2A.6
  Bottom 1.016: IC4.6 127.89,14.45 125.06,17.28 v124.39,17.28 v124.38,17.27
ISENA1  (via drill 0.5)
  Top 0.406: v124.38,63.31 v124.38,63.32 M1A.6
  Bottom 1.016: IC5.6 127.89,60.48 125.06,63.32 v124.39,63.32 v124.38,63.31
ISENA-1
  Top 1.27: R1.2 R2.2
  Bottom 1.27: M1.6 85.41,57.15 R1.2
ISENA-2
  Top 1.27: R7.2 R8.2
  Bottom 1.27: M2.6 85.72,17.78 R8.2
ISENB
  Top 0.406: 129.86,22.07 IC4.9 | M2A.9 126.56,19.23 126.59,19.21
  Top 1.016: 129.86,22.07 127,19.21 126.59,19.21
ISENB1
  Top 0.406: 129.86,68.1 IC5.9 | M1A.9 126.56,65.27 126.59,65.25
  Top 1.016: 129.86,68.1 127,65.25 126.59,65.25
ISENB-1
  Top 1.27: R4.2 R3.2
  Bottom 1.27: M1.9 85.72,64.77 R3.2
ISENB-2
  Top 1.27: R9.2 R10.2
  Bottom 1.27: M2.9 85.41,25.4 R10.2
LED1
  Bottom 0.61: ERR1.A 57.15,73.66 R6.1
LED2
  Bottom 0.61: R5.1 27.94,65.41 ACT(DEC).A
LED3
  Bottom 0.61: ERR2.A 57.15,34.29 R12.1
LED4
  Bottom 0.61: R11.1 4.13,61.28 ACT(RA).A
M0-1  (via drill 0.7)
  Top 0.61: IC1.3 46.83,11.43 46.04,12.22 v46.04,21.43 | v40.32,30.8 40.32,39.05 46.99,45.72 54.61,45.72 v60.96,52.07
  Bottom 0.61: M1.24 63.5,54.61 v60.96,52.07 | v46.04,21.43 46.04,25.08 v40.32,30.8
M0-2
  Bottom 0.61: M2.24 65.09,15.24 64.29,16.03 55.72,16.03 53.98,17.78 43.18,17.78 39.37,13.97 IC1.37
M2-1  (via drill 0.7)
  Top 0.61: IC1.4 48.26,13.97 47.31,14.92 v47.31,22.54 | v41.75,31.11 41.75,39.05 45.88,43.18 56.52,43.18 v62.23,48.9
  Bottom 0.61: M1.26 64.45,49.53 63.82,48.9 v62.23,48.9 | v47.31,22.54 47.31,25.56 v41.75,31.11
M2-2
  Bottom 0.61: M2.26 35.4,10.16 32.38,13.18 32.38,14.76 34.13,16.51 IC1.36
MCLR
  Bottom 0.61: IC2.4 10.48,29.21 9.21,30.48 5.4,30.48 4.13,29.21 4.13,24.45 | 4.13,24.45 2.37,22.68 ICSP.1 | R18.1 4.13,24.45
MISO
  Bottom 0.61: IC1.7 50.8,21.59 49.85,22.54 49.85,24.45 50.8,25.4 53.66,25.4 55.24,26.99 58.74,26.99 61.28,24.45 PROG.1
MODE0
  Top 0.406: M2A.24 118.07,16.63 116.68,15.24 116.68,13.65 IC4.24
MODE1
  Top 0.406: M2A.25 118.38,15.98 117.32,14.92 117.32,11.75 IC4.25
MODE2
  Top 0.406: M2A.26 118.68,15.33 117.95,14.61 117.95,9.84 IC4.26
MODE3
  Top 0.406: M1A.24 118.07,62.67 116.68,61.28 116.68,59.69 IC5.24
MODE4
  Top 0.406: M1A.25 118.38,62.02 117.32,60.96 117.32,57.78 IC5.25
MODE5
  Top 0.406: M1A.26 118.68,61.37 117.95,60.64 117.95,55.88 IC5.26
MOSI
  Bottom 0.61: IC1.6 56.83,19.05 PROG.4
N$1
  Bottom 0.61: IC2.9 27.46,41.91 30,39.37 30,34.77 C18.1
PWRLED
  Bottom 0.61: PWR.A 22.86,56.04 25.56,58.74 R14.2
RESET
  Top 0.61: PROG.5 56.2,23.81 53.34,26.67 IC1.9
  Bottom 0.61: IC1.9 50.48,26.67 48.74,24.92 48.74,21.75 45.88,18.89 42.23,18.89 | 42.23,18.89 38.58,15.24 35.24,15.24 R20.1 | 42.23,18.89 38.26,22.86 34.29,22.86 30,27.15 30,31.27 C18.2
RX(BTH)  (via drill 0.7)
  Top 0.61: IC1.11 49.85,31.75 v47.31,29.21 | R16.1 27.62,46.99 32.07,51.44 32.07,62.87 40.96,71.75 v46.04,71.75
  Bottom 0.61: v47.31,29.21 38.42,38.1 35.56,38.1 26.67,46.99 R16.1 | BLUETOOTH->.4 v46.04,71.75
RX(USB)
  Bottom 0.61: IC2.12 8.89,41.91 9.84,42.86 9.84,45.4 12.7,48.26 16.51,48.26 R16.2
SCLK
  Top 0.61: IC1.8 45.24,24.13 44.45,23.34 44.45,12.38 39.69,7.62 34.92,7.62 R13.1
  Bottom 0.61: IC1.8 54.29,24.13 55.56,25.4 56.83,25.4 PROG.3
STATLED
  Bottom 0.61: STATUS.A 17.78,51.44 20.32,48.9 20.32,46.83 19.21,45.72 13.49,45.72 11.75,43.97 11.75,40.16 13.81,38.1 16.51,38.1 17.78,39.37 26.83,39.37 27.78,38.42 27.78,23.34 R13.2
STEP
  Top 0.406: M2A.22 115.88,17.93 IC4.22
STEP1
  Top 0.406: M1A.22 115.88,63.97 IC5.22
STEP-1  (via drill 0.7)
  Top 0.61: v53.34,4.76 53.02,5.08 29.84,5.08 23.81,11.11 23.81,16.51 33.34,26.04 33.34,32.38 35.24,34.29 IC1.29
  Bottom 0.61: M1.22 68.58,59.69 74.61,53.66 74.61,7.94 68.58,1.91 55.24,1.91 53.34,3.81 v53.34,4.76
STEP-2  (via drill 0.7)
  Top 0.61: IC1.14 v46.99,34.29
  Bottom 0.61: M2.22 66.99,20.32 59.37,27.94 50.8,27.94 46.99,31.75 v46.99,34.29
TX(BTH)  (via drill 0.7)
  Top 0.61: IC1.10 49.21,29.21 v47.31,27.3 | R15.1 33.34,51.12 33.34,62.55 40.96,70.17 47.94,70.17 52.07,74.3 BLUETOOTH->.3 52.39,74.3
  Bottom 0.61: v47.31,27.3 46.04,28.57 46.04,28.89 39.37,35.56 35.56,35.56 R15.1
TX(USB)
  Bottom 0.61: IC2.10 R15.2
USBLED
  Top 0.61: R19.1 4.13,39.85 3.49,40.48 USB.A
USBOSC1
  Top 0.61: IC2.2 15.88,24.13 20.95,29.21 X2.1 21.27,30.48 C15.1
USBOSC2
  Top 0.61: IC2.3 16.83,26.67 19.37,29.21 19.37,33.66 X2.2 C14.1
USBSTAT
  Top 0.61: IC2.16 7.3,31.75 6.99,32.07 R19.2
V3P1
  Top 0.406: M1A.15 119.46,68.5 119.22,68.74 119.22,72.94 | IC5.15 119.22,76.52 119.22,73.66 119.22,72.94 | C6.1 119.22,72.94
V3P3
  Top 0.406: M2A.15 119.46,22.47 119.22,22.7 119.22,26.91 | IC4.15 119.22,30.48 119.22,27.94 119.22,26.91 | C2.1 119.22,26.91
V+  (via drill 0.7)
  Top 1.27: M1.4 v78.11,52.07 | M2.11 v78.11,30.48
  Bottom 0.61: IC3.3 47.31,67.63 48.58,68.9 56.2,68.9 57.15,69.85 63.5,69.85 64.77,68.58 64.77,66.99 65.72,66.04 78.11,66.04
  Bottom 0.813: C10.1 90.49,76.2 89.22,76.2
  Bottom 1.27: C4.+ 86.68,72.71 83.82,69.85 M1.11 80.96,69.85 78.11,66.99 78.11,66.04 v78.11,52.07 v78.11,30.48 78.11,15.24 80.64,12.7 M2.4 84.14,12.7 86.04,10.79 88.9,10.79 C8.+
  Bottom 1.676: C4.+ 86.68,73.98 88.9,76.2 89.22,76.2 89.22,77.79 D1.C
VBUS
  Bottom 0.61: USB->.VBUS 14.14,9.22 D2.A
VCP
  Top 0.305: 128.09,8.49 C3.2 | 128.09,8.91 128.09,8.49 | 128.09,8.49 C3.2
  Top 0.406: M2A.3 126.43,15.33 127.16,14.61 127.16,9.84 128.09,8.91 IC4.3
VCP1
  Top 0.305: 128.09,54.53 C7.2 | 128.09,54.95 128.09,54.53 | 128.09,54.53 C7.2
  Top 0.406: M1A.3 126.43,61.37 127.16,60.64 127.16,55.88 128.09,54.95 IC5.3
VIN
  Top 1.676: J1.PWR 92.71,78.38 D1.A
VMA  (via drill 0.5)
  Top 0.406: v124.38,15.98 M2A.4
  Bottom 1.016: IC4.4 128.27,9.37 126.21,11.43 126.21,14.15 v124.38,15.98
VMA1  (via drill 0.5 pad 0.81)
  Top 0.406: v124.38,62.01 v124.38,62.02 M1A.4
  Bottom 1.016: IC5.4 128.27,55.4 126.21,57.47 126.21,60.19 v124.38,62.01
VMB
  Top 0.406: M2A.11 126.59,20.53 | 129.62,27.15 IC4.11
  Top 1.016: 126.59,20.53 127.79,21.74 127.79,25.32 129.62,27.15
VMB1
  Top 0.406: M1A.11 126.59,66.57 | 129.62,73.18 IC5.11
  Top 1.016: 126.59,66.57 127.79,67.78 127.79,71.36 129.62,73.18
VPIC
  Top 0.61: IC2.1 15.24,18.89 D2.C 15.72,14.29 17.78,12.22 17.78,3.17 15.88,1.27 3.33,1.27 1.75,2.86 1.75,12.54 R18.2
  Bottom 0.61: ICSP.2 3.26,21.18 5.08,19.37 R18.2 | C17.1 D2.C
VUSB
  Top 0.61: IC2.17 C13.2

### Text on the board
Top: Complete | Kit PCB
tNames: Thomas Carpenter (2012) | GND | 3v3 | BRef | !Rst | ARef | !Slp | VMB | !Err | B1 | 12v (4A Max) | Dcy | IsB | Dir | B2 | !EN | A2 | Stp | IsA | A1 | S0 | VMA | A1 | S1 | VCP | S2 | A2 | CP2 | !Home | CP1 | B2 | GND | B1 | A1 | A2 | GND | 3v3 | B2 | BRef | !Rst | B1 | ARef | !Slp | VMB | !Err | B1 | Dcy | IsB | Dir | B2 | !EN | Stp | A2 | IsA | A1 | S0 | V3.0-Kit | VMA | S1 | AstroEQ | VCP | S2 | CP2 | Controller | !Home | CP1 | GND

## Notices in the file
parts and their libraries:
SparkFun: Licensing: CC v3.0 Share-Alike You are welcome to use this library for commercial purposes.
